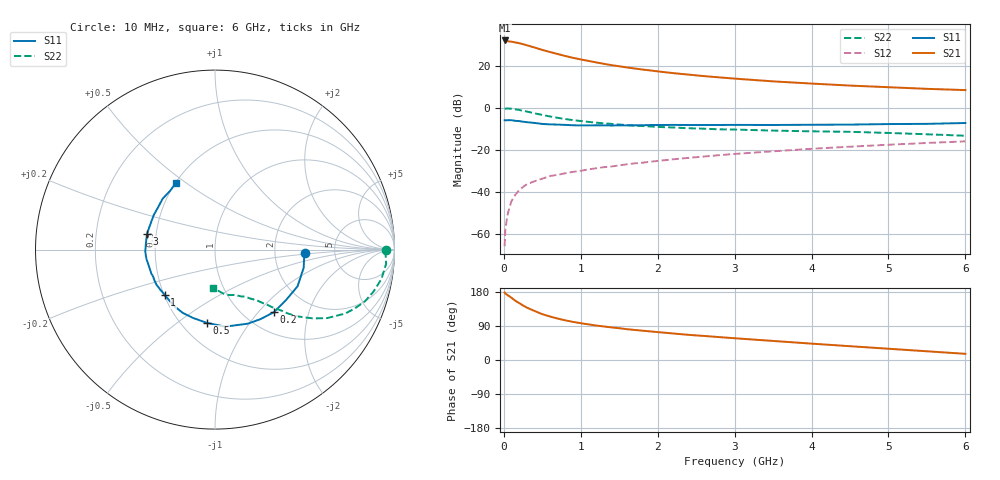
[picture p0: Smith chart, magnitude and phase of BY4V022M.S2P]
! SIEMENS Small Signal Semiconductors
! BFY420
! Si NPN RF SIEGET Grounded Emitter Transistor in MICRO-X
! VCE = 4 V  IC = 22 mA
! Common Emitter S-Parameters:  October  1996
# GHz  S  MA  R  50
!  f  S11  S21  S12  S22
! GHz  MAG  ANG  MAG  ANG  MAG  ANG  MAG  ANG
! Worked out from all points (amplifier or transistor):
!   36 points, 10 MHz to 6 GHz, reference 50 ohm
!   highest |S21| = 32.1 dB at 10 MHz (marker M1)
!   |S21| within 3 dB of that: start of sweep to 365.9 MHz
!   unconditionally stable (mu >= 1): start of sweep to 17.93 MHz; 1.938 GHz to end of sweep
!   at 250 MHz: K = 0.33, MSG = 34.0 dB, |S12| = -37.8 dB
!   at 1.4 GHz: K = 0.92, MSG = 24.2 dB, |S12| = -28.0 dB
!   at 6 GHz: K = 1.06, MAG = 10.8 dB, |S12| = -16.1 dB
!   S11 on the Smith chart (normalised r, x): 10 MHz: 3.00, -0.17; 200 MHz: 1.35, -1.22; 500 MHz: 0.66, -0.65; 1 GHz: 0.50, -0.30; 3 GHz: 0.44, +0.09; 6 GHz: 0.50, +0.46
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0.01  0.5019 -2.4  40.05 178.0  0.0005 51.5  0.9513 -0.3
0.02  0.4983 -4.7  39.5 175.3  0.0013 69.9  0.9503 -1.3
0.1  0.5033 -24.0  37.47 164.2  0.006 75.2  0.9418 -10.0
0.15  0.4855 -35.3  35.94 156.2  0.0084 71.1  0.914 -14.8
0.2  0.4791 -46.6  34.47 150.2  0.0109 70.8  0.884 -19.0
0.25  0.4629 -56.9  32.62 143.7  0.0129 68.1  0.8443 -22.9
0.3  0.4512 -66.2  30.77 138.2  0.0149 66.5  0.8086 -26.1
0.4  0.4329 -82.6  27.18 129.3  0.0177 63.4  0.7339 -31.3
0.5  0.4101 -96.6  23.82 120.9  0.0204 61.3  0.6704 -34.9
0.6  0.4001 -107.7  21.25 114.8  0.0235 60.2  0.6175 -37.6
0.7  0.3956 -117.0  19.02 109.3  0.0251 60.1  0.573 -39.9
0.8  0.3886 -125.5  17.04 104.6  0.0274 58.8  0.5357 -41.4
1  0.3773 -138.0  14.11 97.1  0.0313 59.4  0.4816 -43.6
1.1  0.3778 -143.8  13.04 94.0  0.0337 59.7  0.4591 -44.9
1.3  0.379 -152.5  11.11 88.5  0.0382 60.2  0.424 -46.5
1.6  0.3785 -162.6  9.097 81.3  0.0448 60.2  0.3841 -49.2
2.2  0.3886 -178.3  6.667 70.0  0.0588 58.8  0.3371 -54.1
3  0.3887 166.9  4.932 57.4  0.079 55.0  0.3012 -60.2
3.5  0.3871 158.1  4.241 50.3  0.0913 51.7  0.2845 -64.1
4.5  0.3954 143.1  3.365 36.4  0.1175 44.3  0.2658 -72.6
5.5  0.4117 127.6  2.813 23.0  0.1443 35.5  0.2322 -84.7
6  0.4315 120.1  2.628 16.3  0.1574 30.9  0.2144 -92.5
